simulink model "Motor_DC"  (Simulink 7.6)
settings: Solver=ode23tb  StartTime=0.0  StopTime=10.0  RelTol=1e-3
StopFcn:
  | load Ia_W.mat
  | plot(x(1,:), x(2,:),x(1,:), x(3,:))
  | grid
  | title('Courant armature et vitesse de rotation (rad/s)')
  | xlabel('temps')
  | 
  | delete *.mat, clear all
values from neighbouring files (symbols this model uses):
  A = [1+j -(1-j);1 -2/(1-j)]    [systeme_AX_B_phaseurs.m]
  N = 50;')    [Prog_callbacks.m]    (also in _startup.m = 0.001'))
undefined symbols (not defined in the file or in its folder): constant, Torque
libraries: powerlib x9, simulink x1, powerlib_extras x1

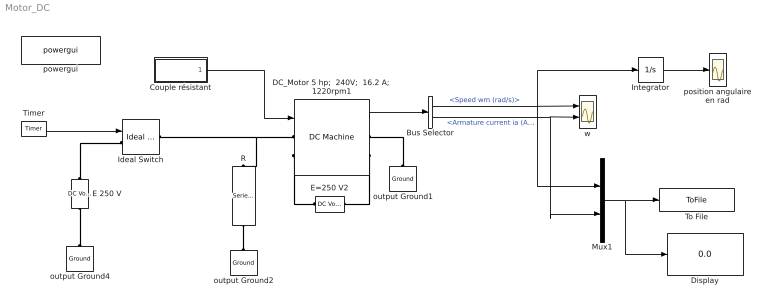
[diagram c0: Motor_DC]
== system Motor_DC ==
  Bus Selector : BusSelector  OutputSignals=Speed wm (rad/s),Armature current ia (A)
  Couple résistant : Subsystem
  DC_Motor 5 hp;  240V;  16.2 A;  1220rpm1 : powerlib/Machines/DC Machine  DialogController=POWERSYS.PowerSysDialog  SystemSampleTime=-1  PresetModel=No  MechanicalLoad=Torque TL  FieldType=Wound  ShowDetailedParameters=on  RLa="[ 0.6  0.012]"  RLf="[ 240  120]"  Laf=1.8  MachineConstant=Torque constant (N.m/A)  Ke=1.8  Kt=1.8  J=1  Bm=0  Tf=0  w0=0  Ifinit=1  TsPowergui=0  TsBlock=-1
  Display : Display
  E 250 V : powerlib/Electrical Sources/DC Voltage Source  Description=source block  DialogController=POWERSYS.PowerSysDialog  SystemSampleTime=-1  Amplitude=240  Measurements=None
  E=250 V2 : powerlib/Electrical Sources/DC Voltage Source  Description=source block  DialogController=POWERSYS.PowerSysDialog  SystemSampleTime=-1  Amplitude=240  Measurements=None
  Ideal Switch : powerlib/Power Electronics/Ideal Switch  DialogController=POWERSYS.PowerSysDialog  SystemSampleTime=-1  Ron=1e-4  Lon=10e-6  IC=0  Rs=inf  Cs=0  Measurements=off
  Integrator : Integrator
  Mux1 : Mux  Inputs=2
  R : powerlib/Elements/Series RLC Branch  DialogController=POWERSYS.PowerSysDialog  PhysicalDomain=powersysdomain  SubClassName=unknown  LeftPortType=p1  RightPortType=p1  LConnTagsString=__new0  RConnTagsString=__new0  BranchType=R  Resistance=1e6  Inductance=1e-3  SetiL0=off  InitialCurrent=0  Capacitance=1e-6  Setx0=off  InitialVoltage=0  Measurements=None
  Timer : powerlib_extras/Control  Blocks/Timer  DialogController=POWERSYS.PowerSysDialog  SystemSampleTime=-1  t=[0 1]  e=[0 1 ]
  To File : ToFile  Filename=Ia_W  MatrixName=x
  output Ground1 : powerlib/Elements/Ground  DialogController=POWERSYS.PowerSysDialog  PhysicalDomain=powersysdomain  SubClassName=unknown  LeftPortType=p1  RightPortType=p1  LConnTagsString=a
  output Ground2 : powerlib/Elements/Ground  DialogController=POWERSYS.PowerSysDialog  PhysicalDomain=powersysdomain  SubClassName=unknown  LeftPortType=p1  RightPortType=p1  LConnTagsString=a
  output Ground4 : powerlib/Elements/Ground  DialogController=POWERSYS.PowerSysDialog  PhysicalDomain=powersysdomain  SubClassName=unknown  LeftPortType=p1  RightPortType=p1  LConnTagsString=a
  position angulaire en rad : Scope
  powergui : powerlib/powergui  Priority=2  SystemSampleTime=-1  SimulationMode=Continuous  SampleTime=0  frequency=60  SPID=off  DisableSnubberDevices=off  DisableRonSwitches=off  DisableVfSwitches=off  SwTol=0  Interpol=off  frequencyindice=0  echomessages=off  HookPort=off  DisplayEquations=off  FunctionMessages=off  EnableUseOfTLC=off  x0status=blocks  RestoreLinks=warning  ResistiveCurrentMeasurement=off  Frange=logspace(0,3,50)  Ylog=off  Xlog=off  ShowGrid=off  save=off  variable=ZData  ZoomFFT=on  StartTime=0.0  cycles=1  DisplayStyle=off  fundamental=60  FreqAxis=off  MaxFrequency=1000  frequencyindicesteady=1  RmsSteady=1  display=off  Ts=0  methode=off
  w : Scope  NumInputPorts=2
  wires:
  Timer/1 -> Ideal Switch/1
  DC_Motor 5 hp;  240V;  16.2 A;  1220rpm1/1 -> Bus Selector/1
  Bus Selector/1 -> w/1, Integrator/1, Mux1/1  "<Speed wm (rad/s)>"
  Couple résistant/1(C) -> DC_Motor 5 hp;  240V;  16.2 A;  1220rpm1/1
  Bus Selector/2 -> w/2, Mux1/2  "<Armature current ia (A)>"
  Integrator/1 -> position angulaire en rad/1
  Mux1/1 -> To File/1, Display/1
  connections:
  E 250 V/LConn1 -- output Ground4/LConn1
  E 250 V/RConn1 -- Ideal Switch/LConn1
  DC_Motor 5 hp;  240V;  16.2 A;  1220rpm1/LConn1 -- Ideal Switch/RConn1 -- R/LConn1
  output Ground1/LConn1 -- DC_Motor 5 hp;  240V;  16.2 A;  1220rpm1/RConn1
  E=250 V2/RConn1 -- DC_Motor 5 hp;  240V;  16.2 A;  1220rpm1/LConn2
  E=250 V2/LConn1 -- DC_Motor 5 hp;  240V;  16.2 A;  1220rpm1/RConn2
  R/RConn1 -- output Ground2/LConn1

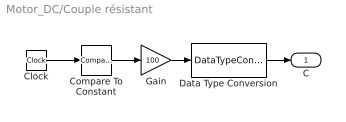
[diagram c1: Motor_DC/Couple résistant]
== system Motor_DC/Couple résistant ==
  Clock : Clock
  Compare To Constant : simulink/Logic and Bit Operations/Compare To Constant  SystemSampleTime=-1  relop=>=  const=5  LogicOutDataTypeMode=uint8
  Data Type Conversion : DataTypeConversion  OutDataTypeStr=double
  Gain : Gain  Gain=100
  C : Outport
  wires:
  Compare To Constant/1 -> Gain/1
  Clock/1 -> Compare To Constant/1
  Gain/1 -> Data Type Conversion/1
  Data Type Conversion/1 -> C/1
